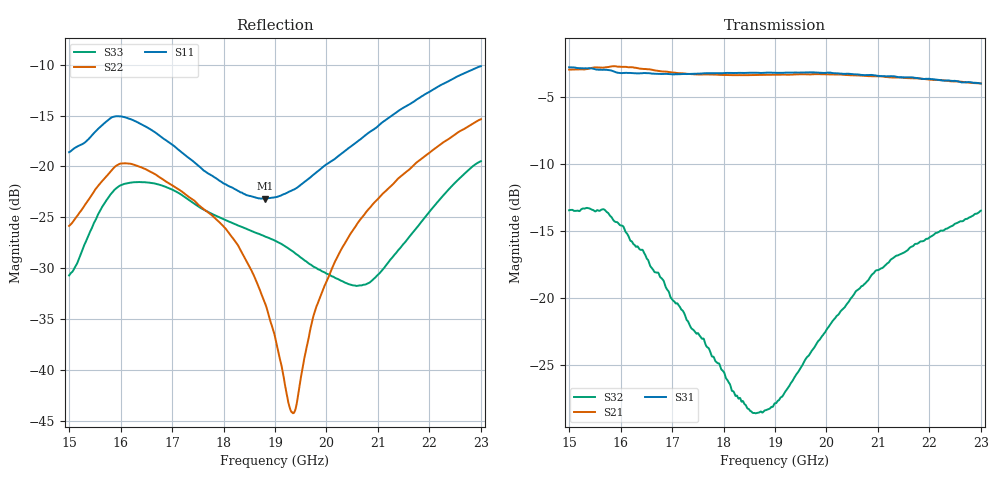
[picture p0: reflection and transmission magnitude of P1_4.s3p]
!The following data was pulled from an Agilent PNA
!This sNp file was generated from the data in the RF Test software
!NOTE:  Smoothing/Math/Corrections applied on any given trace ARE included in the data saved here
# MHz S dB R 50
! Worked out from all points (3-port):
!   1601 points, 15 GHz to 23 GHz, reference 50 ohm
!   strongest paths, dB at 15 GHz, 17 GHz, 19 GHz, 21 GHz, 23 GHz:
!     S31: -2.8, -3.3, -3.2, -3.4, -4.0
!     S21: -2.9, -3.1, -3.3, -3.4, -4.0
!     S32: -13.4, -20.1, -27.8, -17.9, -13.5
!   lowest |S11| = -23.2 dB at 18.8 GHz (marker M1), VSWR 1.15, Z = 51.2 - j6.94 ohm
!   |S11| at or under -10 dB: start of sweep to end of sweep
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15000  -18.60 62.8  -2.97 -171.3  -2.84 -171.9
       -2.94 -171.0  -25.84 106.0  -13.48 148.3
       -2.76 -171.6  -13.44 148.4  -30.71 91.9
15395  -17.22 63.1  -2.86 -176.2  -2.96 -178.6
       -2.85 -176.1  -23.15 101.0  -13.41 138.2
       -2.84 -178.4  -13.30 138.3  -26.55 82.0
15475  -16.77 62.1  -2.84 -177.5  -3.00 -10.4
       -2.79 -177.4  -22.54 98.4  -13.52 135.4
       -2.87 10.7  -13.44 135.2  -25.64 78.9
15605  -16.12 58.9  -2.81 -137.2  -3.03 178.2
       -2.78 -10.3  -21.67 93.9  -13.51 130.6
       -2.95 178.4  -13.45 130.9  -24.36 72.6
15690  -15.73 56.3  -2.77 179.0  -3.07 176.8
       -2.78 179.2  -21.16 90.9  -13.53 126.5
       -2.95 177.1  -13.40 126.5  -23.61 67.8
18800  -23.18 -76.5  -3.39 136.9  -3.23 137.6
       -3.32 136.4  -33.37 14.7  -28.35 -5.3
       -3.18 136.6  -28.38 -5.7  -26.87 -31.3
19000  -23.04 -88.6  -3.36 134.1  -3.19 134.7
       -3.32 133.6  -36.72 22.5  -27.84 -19.7
       -3.17 133.6  -27.84 -20.4  -27.30 -36.6
19365  -22.28 -109.9  -3.31 128.8  -3.16 129.0
       -3.30 128.6  -44.21 94.4  -25.97 -42.1
       -3.16 128.4  -25.98 -42.4  -28.42 -48.6
20465  -18.08 -154.1  -3.31 111.6  -3.25 111.2
       -3.36 111.9  -26.63 147.2  -20.10 -87.5
       -3.25 111.5  -20.05 -87.6  -31.61 -108.2
23000  -10.15 154.3  -3.99 73.5  -3.97 73.6
       -3.97 74.0  -15.37 123.5  -13.44 -143.3
       -3.98 73.6  -13.47 -143.7  -19.49 144.0
